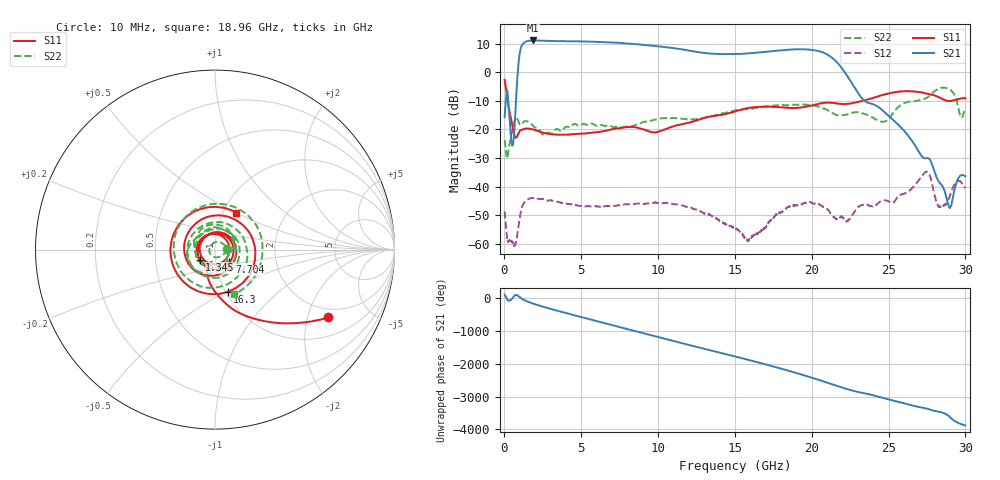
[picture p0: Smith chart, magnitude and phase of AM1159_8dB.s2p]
!Keysight Technologies,N5245B,MY58422270,A.16.20.02
!Date: Tuesday, December 10, 2024 23:28:17
!Correction: S11(C  2-Port  )
!S21(C  2-Port  )
!S12(C  2-Port  )
!S22(C  2-Port  )
!S2P File: Measurements: S11, S21, S12, S22:
# Hz S  dB  R 50
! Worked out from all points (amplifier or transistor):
!   6401 points, 10 MHz to 30 GHz, reference 50 ohm
!   highest |S21| = 11.1 dB at 1.856 GHz (marker M1)
!   |S21| within 3 dB of that: 1.051 GHz to 11.42 GHz (10.37 GHz wide, 166 % of centre)
!   unconditionally stable (mu >= 1): start of sweep to end of sweep
!   at 5.005 GHz: K = 30.77, MAG = 10.9 dB, |S12| = -46.8 dB
!   at 15.01 GHz: K = 116.45, MAG = 6.8 dB, |S12| = -54.5 dB
!   at 30 GHz: K = 2898.38, MAG = -35.6 dB, |S12| = -40.5 dB
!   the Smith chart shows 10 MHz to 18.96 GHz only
!   S11 on the Smith chart (normalised r, x): 10 MHz: 1.65, -2.71; 1.345 GHz: 0.84, -0.10; 7.704 GHz: 1.16, -0.17; 16.3 GHz: 1.02, -0.51; 18.96 GHz: 1.15, +0.50
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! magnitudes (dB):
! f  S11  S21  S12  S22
! 10 MHz  -2.7  -15.7  -48.6  -23.7
! 202.1 MHz  -9.7  -7.2  -58.9  -29.8
! 544.2 MHz  -19.7  -25.4  -59.7  -19.3
! 975.3 MHz  -20.7  6.0  -51.5  -18.0
! 1.345 GHz  -19.8  10.6  -45.3  -17.1
! 1.856 GHz  -20.0  11.1  -44.0  -18.7
! 2.573 GHz  -21.2  11.0  -44.5  -21.9
! 5.01 GHz  -21.5  10.8  -46.8  -18.3
! 7.704 GHz  -19.4  10.2  -46.3  -19.3
! 10.01 GHz  -20.8  9.1  -45.7  -16.3
! 15.01 GHz  -13.7  6.4  -54.5  -13.4
! 16.3 GHz  -12.2  6.8  -56.9  -12.6
! 18.96 GHz  -12.5  8.0  -46.5  -11.4
! 20 GHz  -11.6  7.8  -45.7  -11.5
! 22.3 GHz  -11.1  -1.2  -52.1  -14.8
! 23.18 GHz  -10.2  -8.6  -46.6  -14.2
! 25 GHz  -7.4  -15.3  -45.2  -16.4
! 27.46 GHz  -7.4  -30.1  -34.7  -9.0
! 28.26 GHz  -8.7  -38.2  -46.9  -5.7
! 28.96 GHz  -10.1  -47.3  -43.9  -5.9
! 29.7 GHz  -9.2  -36.1  -38.4  -15.7
! 30 GHz  -9.1  -36.4  -40.5  -12.5
